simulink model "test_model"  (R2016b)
settings: Solver=VariableStepAuto  StartTime=0.0  StopTime=runtime  RelTol=1e-3
InitFcn:
  | clear mex
  | delete test_model_sfun.mexw64
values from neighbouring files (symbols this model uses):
  Delta_T = cell(1,4)    [modelParameters.m]
  F_D = 0    [modelParameters.m]
  g = 9.81    [modelParameters.m]
  Gamma_H = cell(1,4)    [modelParameters.m]
  have_motor_transient = 1    [modelParameters.m]
  height_controlled_o = (((Rm*If        + (((omega0_o * 2 * Rm * Kv * Kq      * Kd + 1)^2) - 1)/(4* Rm*Kv^2*Kq      * Kd))/Vb)*(Pmax - Pmin) + Pmin)    [modelParameters.m]
  i_0 = cell(1,4)    [modelParameters.m]
  If = 0.3836    [modelParameters.m]
  J = diag([ 0.0130 0.0140 0.0285 ])    [modelParameters.m]
  J_L = m_L/12*diag([y_L^2+z_L^2,x_L^2+z_L^2,x_L^2+y_L^2])    [modelParameters.m]
  J_r = cell(1,4)    [modelParameters.m]
  Jreq = 4.2012e-05    [modelParameters.m]
  Jxx = 0.0130    (= 0.013)    [modelParameters.m]
  Jyy = 0.0140    (= 0.014)    [modelParameters.m]
  Jzz = 0.0285    [modelParameters.m]
  K_d = cell(1,4)    [modelParameters.m]
  K_E = cell(1,4)    [modelParameters.m]
  K_H = cell(1,4)    [modelParameters.m]
  K_Q = cell(1,4)    [modelParameters.m]
  K_T = cell(1,4)    [modelParameters.m]
  K_V = cell(1,4)    [modelParameters.m]
  Kd = 1.4852e-07    [modelParameters.m]
  Ki_mahony = 0.001    [modelParameters.m]
  Kp_mahony = 0.4    [modelParameters.m]
  Kq = 96.3422    [modelParameters.m]
  Kt = 1.2007e-05    [modelParameters.m]
  Kv = 96.3422    [modelParameters.m]
  m = 1.216    [modelParameters.m]
  m_L = 0    [modelParameters.m]
  omega0_o = sqrt((m*g)/(4*Kt))    [modelParameters.m]
  omega1_o = sqrt((m*g)/(4*Kt))    [modelParameters.m]
  omega2_o = sqrt((m*g)/(4*Kt))    [modelParameters.m]
  omega3_o = sqrt((m*g)/(4*Kt))    [modelParameters.m]
  omega_0 = cell(1,4)    [modelParameters.m]
  p0 = 0    [modelParameters.m]
  p_0 = cell(1,4)    [modelParameters.m]
  p_max = cell(1,4)    [modelParameters.m]
  phi0 = 0    [modelParameters.m]
  pitch_o = 0    [modelParameters.m]
  pitchrate_o = 0    [modelParameters.m]
  Pmax = 1    [modelParameters.m]
  Pmin = 0    [modelParameters.m]
  psi0 = 0    [modelParameters.m]
  q0 = 0    [modelParameters.m]
  Q_D = 0    [modelParameters.m]
  r0 = 0    [modelParameters.m]
  R_m = cell(1,4)    [modelParameters.m]
  r_oc = [ 0 ; 0 ; 0 ]    [modelParameters.m]
  r_oL = [0; 0; 0]    [modelParameters.m]
  rhx = 0.16    [modelParameters.m]
  rhy = 0.16    [modelParameters.m]
  rhz = 0.03    [modelParameters.m]
  Rm = 0.235    [modelParameters.m]
  roll_o = 0    [modelParameters.m]
  rollrate_o = 0    [modelParameters.m]
  Tc = 0.04    [modelParameters.m]
  theta0 = 0    [modelParameters.m]
  Tq = 0.005    [modelParameters.m]
  u0 = 0    [modelParameters.m]
  v0 = 0    [modelParameters.m]
  Vb = 11.4    [modelParameters.m]
  w0 = 0    [modelParameters.m]
  x0 = 0    [modelParameters.m]
  x_controlled_o = 0    [modelParameters.m]
  x_o = 0    [modelParameters.m]
  x_vel_o = 0    [modelParameters.m]
  y0 = 0    [modelParameters.m]
  y_controlled_o = 0    [modelParameters.m]
  y_o = 0    [modelParameters.m]
  y_vel_o = 0    [modelParameters.m]
  yaw_controlled_o = 0    [modelParameters.m]
  yaw_o = 0    [modelParameters.m]
  yawrate_o = 0    [modelParameters.m]
  z0 = 0    [modelParameters.m]
  z_o = 0    [modelParameters.m]
  z_vel_o = 0    [modelParameters.m]
undefined symbols (not defined in the file or in its folder): Gamma_Omega, Gamma_T, Ki, Kp, r_h, slope, start, Ts, X0
libraries: simulink x16, Derivative x13, dsparch4 x3, vrlib x2
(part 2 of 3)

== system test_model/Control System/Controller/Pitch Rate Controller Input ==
  note: 1) Add Subsystem or Model blocks as valid variant choices. 2) You cannot connect blocks at this level. At simulation, connectivity is automatically determined, based on the active variant and port name matching.
  pitchrate_error_model : Inport
  pitchrate_model : Inport  Port=2
  Feedback : Subsystem  VariantControl=logAnalysisToggle==0
  pitchrate error : Subsystem  VariantControl=logAnalysisToggle==1
  pitchrate_error : Outport
  pitchrate : Outport  Port=2

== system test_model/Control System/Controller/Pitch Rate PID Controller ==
  pitchrate_error : Inport
  pitchrate : Inport  Port=2
  Add : Sum  Inputs=+-
  Discrete D Controller : Derivative/Discrete D Controller  Kd=Kd  a=a
  Discrete PI Controller : simulink/Continuous/PID Controller  Controller=PI  TimeDomain=Discrete-time  SampleTime=Ts  IntegratorMethod=Forward Euler  FilterMethod=Forward Euler  Form=Parallel  UseFilter=on  ControllerParametersSource=internal  P=Kp  I=Ki  D=0  N=100  InitialConditionSource=internal  InitialConditionForIntegrator=0  InitialConditionForFilter=0  ExternalReset=none  LimitOutput=off  UpperSaturationLimit=inf  LowerSaturationLimit=-inf  LinearizeAsGain=off  AntiWindupMode=none  Kb=1  TrackingMode=off  Kt=1  PParamMin=[]  PParamMax=[]  IParamMin=[]  IParamMax=[]  DParamMin=[]  DParamMax=[]  NParamMin=[]  NParamMax=[]  KbParamMin=[]  KbParamMax=[]  KtParamMin=[]  KtParamMax=[]  POutMin=[]  POutMax=[]  IOutMin=[]  IOutMax=[]  DOutMin=[]  DOutMax=[]  NOutMin=[]  NOutMax=[]  KbOutMin=[]  KbOutMax=[]  KtOutMin=[]  KtOutMax=[]  IntegratorOutMin=[]  IntegratorOutMax=[]  FilterOutMin=[]  FilterOutMax=[]  SumOutMin=[]  SumOutMax=[]  SumI1OutMin=[]  SumI1OutMax=[]  SumI2OutMin=[]  SumI2OutMax=[]  SumI3OutMin=[]  SumI3OutMax=[]  SumDOutMin=[]  SumDOutMax=[]  SaturationOutMin=[]  SaturationOutMax=[]  IntegratorContinuousStateAttributes=''  IntegratorStateMustResolveToSignalObject=off  IntegratorRTWStateStorageClass=Auto  FilterContinuousStateAttributes=''  FilterStateMustResolveToSignalObject=off  FilterRTWStateStorageClass=Auto  DifferentiatorICPrevScaledInput=0  DifferentiatorOutMin=[]  DifferentiatorOutMax=[]
  x_motor_command : Outport
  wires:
  pitchrate/1 -> Discrete D Controller/1
  pitchrate_error/1 -> Discrete PI Controller/1
  Discrete PI Controller/1 -> Add/1
  Discrete D Controller/1 -> Add/2
  Add/1 -> x_motor_command/1

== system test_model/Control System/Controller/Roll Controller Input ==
  note: 1) Add Subsystem or Model blocks as valid variant choices. 2) You cannot connect blocks at this level. At simulation, connectivity is automatically determined, based on the active variant and port name matching.
  roll_error_model : Inport
  roll_angle_model : Inport  Port=2
  Feedback : Subsystem  VariantControl=logAnalysisToggle==0
  roll error : Subsystem  VariantControl=logAnalysisToggle==1
  roll_error : Outport
  roll_angle : Outport  Port=2

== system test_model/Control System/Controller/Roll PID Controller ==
  roll_error : Inport
  roll_angle : Inport  Port=2
  Add : Sum  Inputs=+-
  Discrete D Controller : Derivative/Discrete D Controller  Kd=Kd  a=a
  Discrete PI Controller : simulink/Continuous/PID Controller  Controller=PI  TimeDomain=Discrete-time  SampleTime=Ts  IntegratorMethod=Forward Euler  FilterMethod=Forward Euler  Form=Parallel  UseFilter=on  ControllerParametersSource=internal  P=Kp  I=Ki  D=0  N=100  InitialConditionSource=internal  InitialConditionForIntegrator=0  InitialConditionForFilter=0  ExternalReset=none  LimitOutput=off  UpperSaturationLimit=inf  LowerSaturationLimit=-inf  LinearizeAsGain=off  AntiWindupMode=none  Kb=1  TrackingMode=off  Kt=1  PParamMin=[]  PParamMax=[]  IParamMin=[]  IParamMax=[]  DParamMin=[]  DParamMax=[]  NParamMin=[]  NParamMax=[]  KbParamMin=[]  KbParamMax=[]  KtParamMin=[]  KtParamMax=[]  POutMin=[]  POutMax=[]  IOutMin=[]  IOutMax=[]  DOutMin=[]  DOutMax=[]  NOutMin=[]  NOutMax=[]  KbOutMin=[]  KbOutMax=[]  KtOutMin=[]  KtOutMax=[]  IntegratorOutMin=[]  IntegratorOutMax=[]  FilterOutMin=[]  FilterOutMax=[]  SumOutMin=[]  SumOutMax=[]  SumI1OutMin=[]  SumI1OutMax=[]  SumI2OutMin=[]  SumI2OutMax=[]  SumI3OutMin=[]  SumI3OutMax=[]  SumDOutMin=[]  SumDOutMax=[]  SaturationOutMin=[]  SaturationOutMax=[]  IntegratorContinuousStateAttributes=''  IntegratorStateMustResolveToSignalObject=off  IntegratorRTWStateStorageClass=Auto  FilterContinuousStateAttributes=''  FilterStateMustResolveToSignalObject=off  FilterRTWStateStorageClass=Auto  DifferentiatorICPrevScaledInput=0  DifferentiatorOutMin=[]  DifferentiatorOutMax=[]
  rollrate_setpoint : Outport
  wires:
  roll_angle/1 -> Discrete D Controller/1
  roll_error/1 -> Discrete PI Controller/1
  Discrete PI Controller/1 -> Add/1
  Discrete D Controller/1 -> Add/2
  Add/1 -> rollrate_setpoint/1

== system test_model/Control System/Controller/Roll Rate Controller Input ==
  note: 1) Add Subsystem or Model blocks as valid variant choices. 2) You cannot connect blocks at this level. At simulation, connectivity is automatically determined, based on the active variant and port name matching.
  rollrate_error_model : Inport
  rollrate_model : Inport  Port=2
  Feedback : Subsystem  VariantControl=logAnalysisToggle==0
  rollrate error : Subsystem  VariantControl=logAnalysisToggle==1
  rollrate_error : Outport
  rollrate : Outport  Port=2

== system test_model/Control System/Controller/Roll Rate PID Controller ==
  rollrate_error : Inport
  rollrate : Inport  Port=2
  Add : Sum  Inputs=+-
  Discrete D Controller : Derivative/Discrete D Controller  Kd=Kd  a=a
  Discrete PI Controller : simulink/Continuous/PID Controller  Controller=PI  TimeDomain=Discrete-time  SampleTime=Ts  IntegratorMethod=Forward Euler  FilterMethod=Forward Euler  Form=Parallel  UseFilter=on  ControllerParametersSource=internal  P=Kp  I=Ki  D=0  N=100  InitialConditionSource=internal  InitialConditionForIntegrator=0  InitialConditionForFilter=0  ExternalReset=none  LimitOutput=off  UpperSaturationLimit=inf  LowerSaturationLimit=-inf  LinearizeAsGain=off  AntiWindupMode=none  Kb=1  TrackingMode=off  Kt=1  PParamMin=[]  PParamMax=[]  IParamMin=[]  IParamMax=[]  DParamMin=[]  DParamMax=[]  NParamMin=[]  NParamMax=[]  KbParamMin=[]  KbParamMax=[]  KtParamMin=[]  KtParamMax=[]  POutMin=[]  POutMax=[]  IOutMin=[]  IOutMax=[]  DOutMin=[]  DOutMax=[]  NOutMin=[]  NOutMax=[]  KbOutMin=[]  KbOutMax=[]  KtOutMin=[]  KtOutMax=[]  IntegratorOutMin=[]  IntegratorOutMax=[]  FilterOutMin=[]  FilterOutMax=[]  SumOutMin=[]  SumOutMax=[]  SumI1OutMin=[]  SumI1OutMax=[]  SumI2OutMin=[]  SumI2OutMax=[]  SumI3OutMin=[]  SumI3OutMax=[]  SumDOutMin=[]  SumDOutMax=[]  SaturationOutMin=[]  SaturationOutMax=[]  IntegratorContinuousStateAttributes=''  IntegratorStateMustResolveToSignalObject=off  IntegratorRTWStateStorageClass=Auto  FilterContinuousStateAttributes=''  FilterStateMustResolveToSignalObject=off  FilterRTWStateStorageClass=Auto  DifferentiatorICPrevScaledInput=0  DifferentiatorOutMin=[]  DifferentiatorOutMax=[]
  y_motor_command : Outport
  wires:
  rollrate/1 -> Discrete D Controller/1
  rollrate_error/1 -> Discrete PI Controller/1
  Discrete PI Controller/1 -> Add/1
  Discrete D Controller/1 -> Add/2
  Add/1 -> y_motor_command/1

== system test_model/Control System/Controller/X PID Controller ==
  x_error : Inport
  x_pos : Inport  Port=2
  Add : Sum  Inputs=+-
  Discrete D Controller : Derivative/Discrete D Controller  Kd=Kd  a=a
  Discrete PI Controller : simulink/Continuous/PID Controller  Controller=PI  TimeDomain=Discrete-time  SampleTime=Ts  IntegratorMethod=Forward Euler  FilterMethod=Forward Euler  Form=Parallel  UseFilter=on  ControllerParametersSource=internal  P=Kp  I=Ki  D=0  N=100  InitialConditionSource=internal  InitialConditionForIntegrator=0  InitialConditionForFilter=0  ExternalReset=none  LimitOutput=off  UpperSaturationLimit=inf  LowerSaturationLimit=-inf  LinearizeAsGain=off  AntiWindupMode=none  Kb=1  TrackingMode=off  Kt=1  PParamMin=[]  PParamMax=[]  IParamMin=[]  IParamMax=[]  DParamMin=[]  DParamMax=[]  NParamMin=[]  NParamMax=[]  KbParamMin=[]  KbParamMax=[]  KtParamMin=[]  KtParamMax=[]  POutMin=[]  POutMax=[]  IOutMin=[]  IOutMax=[]  DOutMin=[]  DOutMax=[]  NOutMin=[]  NOutMax=[]  KbOutMin=[]  KbOutMax=[]  KtOutMin=[]  KtOutMax=[]  IntegratorOutMin=[]  IntegratorOutMax=[]  FilterOutMin=[]  FilterOutMax=[]  SumOutMin=[]  SumOutMax=[]  SumI1OutMin=[]  SumI1OutMax=[]  SumI2OutMin=[]  SumI2OutMax=[]  SumI3OutMin=[]  SumI3OutMax=[]  SumDOutMin=[]  SumDOutMax=[]  SaturationOutMin=[]  SaturationOutMax=[]  IntegratorContinuousStateAttributes=''  IntegratorStateMustResolveToSignalObject=off  IntegratorRTWStateStorageClass=Auto  FilterContinuousStateAttributes=''  FilterStateMustResolveToSignalObject=off  FilterRTWStateStorageClass=Auto  DifferentiatorICPrevScaledInput=0  DifferentiatorOutMin=[]  DifferentiatorOutMax=[]
  pitch_setpoint : Outport
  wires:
  x_pos/1 -> Discrete D Controller/1
  x_error/1 -> Discrete PI Controller/1
  Discrete PI Controller/1 -> Add/1
  Discrete D Controller/1 -> Add/2
  Add/1 -> pitch_setpoint/1

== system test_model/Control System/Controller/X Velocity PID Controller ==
  x_vel_error : Inport
  x_vel : Inport  Port=2
  Add : Sum  Inputs=+-
  Discrete D Controller : Derivative/Discrete D Controller  Kd=Kd  a=a
  Discrete PI Controller : simulink/Continuous/PID Controller  Controller=PI  TimeDomain=Discrete-time  SampleTime=Ts  IntegratorMethod=Forward Euler  FilterMethod=Forward Euler  Form=Parallel  UseFilter=on  ControllerParametersSource=internal  P=Kp  I=Ki  D=0  N=100  InitialConditionSource=internal  InitialConditionForIntegrator=0  InitialConditionForFilter=0  ExternalReset=none  LimitOutput=off  UpperSaturationLimit=inf  LowerSaturationLimit=-inf  LinearizeAsGain=off  AntiWindupMode=none  Kb=1  TrackingMode=off  Kt=1  PParamMin=[]  PParamMax=[]  IParamMin=[]  IParamMax=[]  DParamMin=[]  DParamMax=[]  NParamMin=[]  NParamMax=[]  KbParamMin=[]  KbParamMax=[]  KtParamMin=[]  KtParamMax=[]  POutMin=[]  POutMax=[]  IOutMin=[]  IOutMax=[]  DOutMin=[]  DOutMax=[]  NOutMin=[]  NOutMax=[]  KbOutMin=[]  KbOutMax=[]  KtOutMin=[]  KtOutMax=[]  IntegratorOutMin=[]  IntegratorOutMax=[]  FilterOutMin=[]  FilterOutMax=[]  SumOutMin=[]  SumOutMax=[]  SumI1OutMin=[]  SumI1OutMax=[]  SumI2OutMin=[]  SumI2OutMax=[]  SumI3OutMin=[]  SumI3OutMax=[]  SumDOutMin=[]  SumDOutMax=[]  SaturationOutMin=[]  SaturationOutMax=[]  IntegratorContinuousStateAttributes=''  IntegratorStateMustResolveToSignalObject=off  IntegratorRTWStateStorageClass=Auto  FilterContinuousStateAttributes=''  FilterStateMustResolveToSignalObject=off  FilterRTWStateStorageClass=Auto  DifferentiatorICPrevScaledInput=0  DifferentiatorOutMin=[]  DifferentiatorOutMax=[]
  pitch_setpoint : Outport
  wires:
  x_vel/1 -> Discrete D Controller/1
  x_vel_error/1 -> Discrete PI Controller/1
  Discrete PI Controller/1 -> Add/1
  Discrete D Controller/1 -> Add/2
  Add/1 -> pitch_setpoint/1

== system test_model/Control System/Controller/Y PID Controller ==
  y_error : Inport
  y_pos : Inport  Port=2
  Add : Sum  Inputs=+-
  Discrete D Controller : Derivative/Discrete D Controller  Kd=Kd  a=a
  Discrete PI Controller : simulink/Continuous/PID Controller  Controller=PI  TimeDomain=Discrete-time  SampleTime=Ts  IntegratorMethod=Forward Euler  FilterMethod=Forward Euler  Form=Parallel  UseFilter=on  ControllerParametersSource=internal  P=Kp  I=Ki  D=0  N=100  InitialConditionSource=internal  InitialConditionForIntegrator=0  InitialConditionForFilter=0  ExternalReset=none  LimitOutput=off  UpperSaturationLimit=inf  LowerSaturationLimit=-inf  LinearizeAsGain=off  AntiWindupMode=none  Kb=1  TrackingMode=off  Kt=1  PParamMin=[]  PParamMax=[]  IParamMin=[]  IParamMax=[]  DParamMin=[]  DParamMax=[]  NParamMin=[]  NParamMax=[]  KbParamMin=[]  KbParamMax=[]  KtParamMin=[]  KtParamMax=[]  POutMin=[]  POutMax=[]  IOutMin=[]  IOutMax=[]  DOutMin=[]  DOutMax=[]  NOutMin=[]  NOutMax=[]  KbOutMin=[]  KbOutMax=[]  KtOutMin=[]  KtOutMax=[]  IntegratorOutMin=[]  IntegratorOutMax=[]  FilterOutMin=[]  FilterOutMax=[]  SumOutMin=[]  SumOutMax=[]  SumI1OutMin=[]  SumI1OutMax=[]  SumI2OutMin=[]  SumI2OutMax=[]  SumI3OutMin=[]  SumI3OutMax=[]  SumDOutMin=[]  SumDOutMax=[]  SaturationOutMin=[]  SaturationOutMax=[]  IntegratorContinuousStateAttributes=''  IntegratorStateMustResolveToSignalObject=off  IntegratorRTWStateStorageClass=Auto  FilterContinuousStateAttributes=''  FilterStateMustResolveToSignalObject=off  FilterRTWStateStorageClass=Auto  DifferentiatorICPrevScaledInput=0  DifferentiatorOutMin=[]  DifferentiatorOutMax=[]
  roll_setpoint : Outport
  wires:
  y_pos/1 -> Discrete D Controller/1
  y_error/1 -> Discrete PI Controller/1
  Discrete PI Controller/1 -> Add/1
  Discrete D Controller/1 -> Add/2
  Add/1 -> roll_setpoint/1

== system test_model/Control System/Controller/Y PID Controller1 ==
  y_error : Inport
  y_pos : Inport  Port=2
  Add : Sum  Inputs=+-
  Discrete D Controller : Derivative/Discrete D Controller  Kd=Kd  a=a
  Discrete PI Controller : simulink/Continuous/PID Controller  Controller=PI  TimeDomain=Discrete-time  SampleTime=Ts  IntegratorMethod=Forward Euler  FilterMethod=Forward Euler  Form=Parallel  UseFilter=on  ControllerParametersSource=internal  P=Kp  I=Ki  D=0  N=100  InitialConditionSource=internal  InitialConditionForIntegrator=0  InitialConditionForFilter=0  ExternalReset=none  LimitOutput=off  UpperSaturationLimit=inf  LowerSaturationLimit=-inf  LinearizeAsGain=off  AntiWindupMode=none  Kb=1  TrackingMode=off  Kt=1  PParamMin=[]  PParamMax=[]  IParamMin=[]  IParamMax=[]  DParamMin=[]  DParamMax=[]  NParamMin=[]  NParamMax=[]  KbParamMin=[]  KbParamMax=[]  KtParamMin=[]  KtParamMax=[]  POutMin=[]  POutMax=[]  IOutMin=[]  IOutMax=[]  DOutMin=[]  DOutMax=[]  NOutMin=[]  NOutMax=[]  KbOutMin=[]  KbOutMax=[]  KtOutMin=[]  KtOutMax=[]  IntegratorOutMin=[]  IntegratorOutMax=[]  FilterOutMin=[]  FilterOutMax=[]  SumOutMin=[]  SumOutMax=[]  SumI1OutMin=[]  SumI1OutMax=[]  SumI2OutMin=[]  SumI2OutMax=[]  SumI3OutMin=[]  SumI3OutMax=[]  SumDOutMin=[]  SumDOutMax=[]  SaturationOutMin=[]  SaturationOutMax=[]  IntegratorContinuousStateAttributes=''  IntegratorStateMustResolveToSignalObject=off  IntegratorRTWStateStorageClass=Auto  FilterContinuousStateAttributes=''  FilterStateMustResolveToSignalObject=off  FilterRTWStateStorageClass=Auto  DifferentiatorICPrevScaledInput=0  DifferentiatorOutMin=[]  DifferentiatorOutMax=[]
  y_vel_setpoint : Outport
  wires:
  y_pos/1 -> Discrete D Controller/1
  y_error/1 -> Discrete PI Controller/1
  Discrete PI Controller/1 -> Add/1
  Discrete D Controller/1 -> Add/2
  Add/1 -> y_vel_setpoint/1

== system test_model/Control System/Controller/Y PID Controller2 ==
  x_error : Inport
  x_pos : Inport  Port=2
  Add : Sum  Inputs=+-
  Discrete D Controller : Derivative/Discrete D Controller  Kd=Kd  a=a
  Discrete PI Controller : simulink/Continuous/PID Controller  Controller=PI  TimeDomain=Discrete-time  SampleTime=Ts  IntegratorMethod=Forward Euler  FilterMethod=Forward Euler  Form=Parallel  UseFilter=on  ControllerParametersSource=internal  P=Kp  I=Ki  D=0  N=100  InitialConditionSource=internal  InitialConditionForIntegrator=0  InitialConditionForFilter=0  ExternalReset=none  LimitOutput=off  UpperSaturationLimit=inf  LowerSaturationLimit=-inf  LinearizeAsGain=off  AntiWindupMode=none  Kb=1  TrackingMode=off  Kt=1  PParamMin=[]  PParamMax=[]  IParamMin=[]  IParamMax=[]  DParamMin=[]  DParamMax=[]  NParamMin=[]  NParamMax=[]  KbParamMin=[]  KbParamMax=[]  KtParamMin=[]  KtParamMax=[]  POutMin=[]  POutMax=[]  IOutMin=[]  IOutMax=[]  DOutMin=[]  DOutMax=[]  NOutMin=[]  NOutMax=[]  KbOutMin=[]  KbOutMax=[]  KtOutMin=[]  KtOutMax=[]  IntegratorOutMin=[]  IntegratorOutMax=[]  FilterOutMin=[]  FilterOutMax=[]  SumOutMin=[]  SumOutMax=[]  SumI1OutMin=[]  SumI1OutMax=[]  SumI2OutMin=[]  SumI2OutMax=[]  SumI3OutMin=[]  SumI3OutMax=[]  SumDOutMin=[]  SumDOutMax=[]  SaturationOutMin=[]  SaturationOutMax=[]  IntegratorContinuousStateAttributes=''  IntegratorStateMustResolveToSignalObject=off  IntegratorRTWStateStorageClass=Auto  FilterContinuousStateAttributes=''  FilterStateMustResolveToSignalObject=off  FilterRTWStateStorageClass=Auto  DifferentiatorICPrevScaledInput=0  DifferentiatorOutMin=[]  DifferentiatorOutMax=[]
  x_vel_setpoint : Outport
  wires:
  x_pos/1 -> Discrete D Controller/1
  x_error/1 -> Discrete PI Controller/1
  Discrete PI Controller/1 -> Add/1
  Discrete D Controller/1 -> Add/2
  Add/1 -> x_vel_setpoint/1

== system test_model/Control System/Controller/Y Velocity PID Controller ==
  y_error : Inport
  y_pos : Inport  Port=2
  Add : Sum  Inputs=+-
  Discrete D Controller : Derivative/Discrete D Controller  Kd=Kd  a=a
  Discrete PI Controller : simulink/Continuous/PID Controller  Controller=PI  TimeDomain=Discrete-time  SampleTime=Ts  IntegratorMethod=Forward Euler  FilterMethod=Forward Euler  Form=Parallel  UseFilter=on  ControllerParametersSource=internal  P=Kp  I=Ki  D=0  N=100  InitialConditionSource=internal  InitialConditionForIntegrator=0  InitialConditionForFilter=0  ExternalReset=none  LimitOutput=off  UpperSaturationLimit=inf  LowerSaturationLimit=-inf  LinearizeAsGain=off  AntiWindupMode=none  Kb=1  TrackingMode=off  Kt=1  PParamMin=[]  PParamMax=[]  IParamMin=[]  IParamMax=[]  DParamMin=[]  DParamMax=[]  NParamMin=[]  NParamMax=[]  KbParamMin=[]  KbParamMax=[]  KtParamMin=[]  KtParamMax=[]  POutMin=[]  POutMax=[]  IOutMin=[]  IOutMax=[]  DOutMin=[]  DOutMax=[]  NOutMin=[]  NOutMax=[]  KbOutMin=[]  KbOutMax=[]  KtOutMin=[]  KtOutMax=[]  IntegratorOutMin=[]  IntegratorOutMax=[]  FilterOutMin=[]  FilterOutMax=[]  SumOutMin=[]  SumOutMax=[]  SumI1OutMin=[]  SumI1OutMax=[]  SumI2OutMin=[]  SumI2OutMax=[]  SumI3OutMin=[]  SumI3OutMax=[]  SumDOutMin=[]  SumDOutMax=[]  SaturationOutMin=[]  SaturationOutMax=[]  IntegratorContinuousStateAttributes=''  IntegratorStateMustResolveToSignalObject=off  IntegratorRTWStateStorageClass=Auto  FilterContinuousStateAttributes=''  FilterStateMustResolveToSignalObject=off  FilterRTWStateStorageClass=Auto  DifferentiatorICPrevScaledInput=0  DifferentiatorOutMin=[]  DifferentiatorOutMax=[]
  roll_setpoint : Outport
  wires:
  y_pos/1 -> Discrete D Controller/1
  y_error/1 -> Discrete PI Controller/1
  Discrete PI Controller/1 -> Add/1
  Discrete D Controller/1 -> Add/2
  Add/1 -> roll_setpoint/1

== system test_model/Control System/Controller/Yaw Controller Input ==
  note: 1) Add Subsystem or Model blocks as valid variant choices. 2) You cannot connect blocks at this level. At simulation, connectivity is automatically determined, based on the active variant and port name matching.
  yaw_error_model : Inport
  yaw_angle_model : Inport  Port=2
  Feedback : Subsystem  VariantControl=logAnalysisToggle==0
  yaw error : Subsystem  VariantControl=logAnalysisToggle==1
  yaw_error : Outport
  yaw_angle : Outport  Port=2

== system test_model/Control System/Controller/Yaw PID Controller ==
  yaw_error : Inport
  yaw_angle : Inport  Port=2
  Add : Sum  Inputs=+-
  Discrete D Controller : Derivative/Discrete D Controller  Kd=Kd  a=a
  Discrete PI Controller : simulink/Continuous/PID Controller  Controller=PI  TimeDomain=Discrete-time  SampleTime=Ts  IntegratorMethod=Forward Euler  FilterMethod=Forward Euler  Form=Parallel  UseFilter=on  ControllerParametersSource=internal  P=Kp  I=Ki  D=0  N=100  InitialConditionSource=internal  InitialConditionForIntegrator=0  InitialConditionForFilter=0  ExternalReset=none  LimitOutput=off  UpperSaturationLimit=inf  LowerSaturationLimit=-inf  LinearizeAsGain=off  AntiWindupMode=none  Kb=1  TrackingMode=off  Kt=1  PParamMin=[]  PParamMax=[]  IParamMin=[]  IParamMax=[]  DParamMin=[]  DParamMax=[]  NParamMin=[]  NParamMax=[]  KbParamMin=[]  KbParamMax=[]  KtParamMin=[]  KtParamMax=[]  POutMin=[]  POutMax=[]  IOutMin=[]  IOutMax=[]  DOutMin=[]  DOutMax=[]  NOutMin=[]  NOutMax=[]  KbOutMin=[]  KbOutMax=[]  KtOutMin=[]  KtOutMax=[]  IntegratorOutMin=[]  IntegratorOutMax=[]  FilterOutMin=[]  FilterOutMax=[]  SumOutMin=[]  SumOutMax=[]  SumI1OutMin=[]  SumI1OutMax=[]  SumI2OutMin=[]  SumI2OutMax=[]  SumI3OutMin=[]  SumI3OutMax=[]  SumDOutMin=[]  SumDOutMax=[]  SaturationOutMin=[]  SaturationOutMax=[]  IntegratorContinuousStateAttributes=''  IntegratorStateMustResolveToSignalObject=off  IntegratorRTWStateStorageClass=Auto  FilterContinuousStateAttributes=''  FilterStateMustResolveToSignalObject=off  FilterRTWStateStorageClass=Auto  DifferentiatorICPrevScaledInput=0  DifferentiatorOutMin=[]  DifferentiatorOutMax=[]
  yawrate_setpoint : Outport
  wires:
  yaw_angle/1 -> Discrete D Controller/1
  yaw_error/1 -> Discrete PI Controller/1
  Discrete PI Controller/1 -> Add/1
  Discrete D Controller/1 -> Add/2
  Add/1 -> yawrate_setpoint/1

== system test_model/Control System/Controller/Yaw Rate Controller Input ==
  note: 1) Add Subsystem or Model blocks as valid variant choices. 2) You cannot connect blocks at this level. At simulation, connectivity is automatically determined, based on the active variant and port name matching.
  yawrate_error_model : Inport
  yawrate_model : Inport  Port=2
  Feedback : Subsystem  VariantControl=logAnalysisToggle==0
  yawrate error : Subsystem  VariantControl=logAnalysisToggle==1
  yawrate_error : Outport
  yawrate : Outport  Port=2

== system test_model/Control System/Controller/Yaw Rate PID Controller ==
  yawrate_error : Inport
  yawrate : Inport  Port=2
  Add : Sum  Inputs=+-
  Discrete D Controller : Derivative/Discrete D Controller  Kd=Kd  a=a
  Discrete PI Controller : simulink/Continuous/PID Controller  Controller=PI  TimeDomain=Discrete-time  SampleTime=Ts  IntegratorMethod=Forward Euler  FilterMethod=Forward Euler  Form=Parallel  UseFilter=on  ControllerParametersSource=internal  P=Kp  I=Ki  D=0  N=100  InitialConditionSource=internal  InitialConditionForIntegrator=0  InitialConditionForFilter=0  ExternalReset=none  LimitOutput=off  UpperSaturationLimit=inf  LowerSaturationLimit=-inf  LinearizeAsGain=off  AntiWindupMode=none  Kb=1  TrackingMode=off  Kt=1  PParamMin=[]  PParamMax=[]  IParamMin=[]  IParamMax=[]  DParamMin=[]  DParamMax=[]  NParamMin=[]  NParamMax=[]  KbParamMin=[]  KbParamMax=[]  KtParamMin=[]  KtParamMax=[]  POutMin=[]  POutMax=[]  IOutMin=[]  IOutMax=[]  DOutMin=[]  DOutMax=[]  NOutMin=[]  NOutMax=[]  KbOutMin=[]  KbOutMax=[]  KtOutMin=[]  KtOutMax=[]  IntegratorOutMin=[]  IntegratorOutMax=[]  FilterOutMin=[]  FilterOutMax=[]  SumOutMin=[]  SumOutMax=[]  SumI1OutMin=[]  SumI1OutMax=[]  SumI2OutMin=[]  SumI2OutMax=[]  SumI3OutMin=[]  SumI3OutMax=[]  SumDOutMin=[]  SumDOutMax=[]  SaturationOutMin=[]  SaturationOutMax=[]  IntegratorContinuousStateAttributes=''  IntegratorStateMustResolveToSignalObject=off  IntegratorRTWStateStorageClass=Auto  FilterContinuousStateAttributes=''  FilterStateMustResolveToSignalObject=off  FilterRTWStateStorageClass=Auto  DifferentiatorICPrevScaledInput=0  DifferentiatorOutMin=[]  DifferentiatorOutMax=[]
  yaw_motor_command : Outport
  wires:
  yawrate/1 -> Discrete D Controller/1
  yawrate_error/1 -> Discrete PI Controller/1
  Discrete PI Controller/1 -> Add/1
  Discrete D Controller/1 -> Add/2
  Add/1 -> yaw_motor_command/1

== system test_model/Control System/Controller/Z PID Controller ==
  z_error : Inport
  z_pos : Inport  Port=2
  Add : Sum  Inputs=+-
  Discrete D Controller : Derivative/Discrete D Controller  Kd=Kd  a=a
  Discrete PI Controller : simulink/Continuous/PID Controller  Controller=PI  TimeDomain=Discrete-time  SampleTime=Ts  IntegratorMethod=Forward Euler  FilterMethod=Forward Euler  Form=Parallel  UseFilter=on  ControllerParametersSource=internal  P=Kp  I=Ki  D=0  N=100  InitialConditionSource=internal  InitialConditionForIntegrator=0  InitialConditionForFilter=0  ExternalReset=none  LimitOutput=off  UpperSaturationLimit=inf  LowerSaturationLimit=-inf  LinearizeAsGain=off  AntiWindupMode=none  Kb=1  TrackingMode=off  Kt=1  PParamMin=[]  PParamMax=[]  IParamMin=[]  IParamMax=[]  DParamMin=[]  DParamMax=[]  NParamMin=[]  NParamMax=[]  KbParamMin=[]  KbParamMax=[]  KtParamMin=[]  KtParamMax=[]  POutMin=[]  POutMax=[]  IOutMin=[]  IOutMax=[]  DOutMin=[]  DOutMax=[]  NOutMin=[]  NOutMax=[]  KbOutMin=[]  KbOutMax=[]  KtOutMin=[]  KtOutMax=[]  IntegratorOutMin=[]  IntegratorOutMax=[]  FilterOutMin=[]  FilterOutMax=[]  SumOutMin=[]  SumOutMax=[]  SumI1OutMin=[]  SumI1OutMax=[]  SumI2OutMin=[]  SumI2OutMax=[]  SumI3OutMin=[]  SumI3OutMax=[]  SumDOutMin=[]  SumDOutMax=[]  SaturationOutMin=[]  SaturationOutMax=[]  IntegratorContinuousStateAttributes=''  IntegratorStateMustResolveToSignalObject=off  IntegratorRTWStateStorageClass=Auto  FilterContinuousStateAttributes=''  FilterStateMustResolveToSignalObject=off  FilterRTWStateStorageClass=Auto  DifferentiatorICPrevScaledInput=0  DifferentiatorOutMin=[]  DifferentiatorOutMax=[]
  z_motor_command : Outport
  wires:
  z_pos/1 -> Discrete D Controller/1
  z_error/1 -> Discrete PI Controller/1
  Discrete PI Controller/1 -> Add/1
  Discrete D Controller/1 -> Add/2
  Add/1 -> z_motor_command/1

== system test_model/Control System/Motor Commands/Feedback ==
  z_command_model : Inport
  z_command : Outport
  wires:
  z_command_model/1 -> z_command/1

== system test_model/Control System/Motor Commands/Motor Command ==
  From Workspace5 : FromWorkspace  VariableName=motor_commands  SampleTime=Tq
  z_command : Outport
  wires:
  From Workspace5/1 -> z_command/1

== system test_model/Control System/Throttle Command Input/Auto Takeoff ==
  height_controlled_o : Constant  Value=0.45  SampleTime=Tc
  z_command : Outport
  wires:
  height_controlled_o/1 -> z_command/1

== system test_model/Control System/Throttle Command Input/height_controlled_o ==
  height_controlled_o : Constant  Value=height_controlled_o  SampleTime=Tc
  z_command : Outport
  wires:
  height_controlled_o/1 -> z_command/1

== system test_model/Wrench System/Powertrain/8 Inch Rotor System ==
  M : Inport
  Lambda : Inport  Port=2
  8 Inch Rotor 1 : Subsystem
  8 Inch Rotor 2 : Subsystem
  8 Inch Rotor 3 : Subsystem
  8 Inch Rotor 4 : Subsystem
  Bus Creator : BusCreator  Inputs=8
  Bus Selector : BusSelector  OutputSignals=signal1.alpha_1,signal1.omega_1
  Bus Selector1 : BusSelector  OutputSignals=signal2.alpha_2,signal2.omega_2
  Bus Selector2 : BusSelector  OutputSignals=signal3.alpha_3,signal3.omega_3
  Bus Selector3 : BusSelector  OutputSignals=signal4.alpha_4,signal4.omega_4
  Bus Selector{4..7} (4 alike) : BusSelector  OutputSignals=v_o,Omega
  W_r : Outport
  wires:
  8 Inch Rotor 4/1(F) -> Bus Creator/7  "F_r_4"
  8 Inch Rotor 3/2(Q) -> Bus Creator/6  "Q_r_3"
  8 Inch Rotor 3/1(F) -> Bus Creator/5  "F_r_3"
  8 Inch Rotor 2/2(Q) -> Bus Creator/4  "Q_r_2"
  8 Inch Rotor 2/1(F) -> Bus Creator/3  "F_r_2"
  8 Inch Rotor 4/2(Q) -> Bus Creator/8  "Q_r_4"
  8 Inch Rotor 1/2(Q) -> Bus Creator/2  "Q_r_1"
  8 Inch Rotor 1/1(F) -> Bus Creator/1  "F_r_1"
  Bus Creator/1 -> W_r/1
  Bus Selector/1 -> 8 Inch Rotor 1/1(alpha)  "<alpha_1>"
  Bus Selector/2 -> 8 Inch Rotor 1/2(omega)  "<omega_1>"
  Bus Selector4/1 -> 8 Inch Rotor 1/3(v)  "<v_o>"
  Bus Selector4/2 -> 8 Inch Rotor 1/4(Omega)  "<Omega>"
  Bus Selector1/1 -> 8 Inch Rotor 2/1(alpha)  "<alpha_2>"
  Bus Selector1/2 -> 8 Inch Rotor 2/2(omega)  "<omega_2>"
  Bus Selector5/1 -> 8 Inch Rotor 2/3(v)  "<v_o>"
  Bus Selector5/2 -> 8 Inch Rotor 2/4(Omega)  "<Omega>"
  Bus Selector2/1 -> 8 Inch Rotor 3/1(alpha)  "<alpha_3>"
  Bus Selector2/2 -> 8 Inch Rotor 3/2(omega)  "<omega_3>"
  Bus Selector7/1 -> 8 Inch Rotor 3/3(v)  "<v_o>"
  Bus Selector7/2 -> 8 Inch Rotor 3/4(Omega)  "<Omega>"
  Bus Selector3/1 -> 8 Inch Rotor 4/1(alpha)  "<alpha_4>"
  Bus Selector3/2 -> 8 Inch Rotor 4/2(omega)  "<omega_4>"
  Bus Selector6/1 -> 8 Inch Rotor 4/3(v)  "<v_o>"
  Bus Selector6/2 -> 8 Inch Rotor 4/4(Omega)  "<Omega>"
  Lambda/1 -> Bus Selector4/1, Bus Selector5/1, Bus Selector7/1, Bus Selector6/1
  M/1 -> Bus Selector/1, Bus Selector1/1, Bus Selector2/1, Bus Selector3/1

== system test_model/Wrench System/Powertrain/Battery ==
  Ramp : Subsystem
  V : Outport
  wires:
  Ramp/1(Out1) -> V/1

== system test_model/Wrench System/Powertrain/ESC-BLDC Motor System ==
  P : Inport
  V_b : Inport  Port=2
  Bus Creator{,1..3} (4 alike) : BusCreator  Inputs=2
  Bus Creator4 : BusCreator  Inputs=4
  Demux : Demux
  ESC and BLDC Motor 1 : Subsystem
  ESC and BLDC Motor 2 : Subsystem
  ESC and BLDC Motor 3 : Subsystem
  ESC and BLDC Motor 4 : Subsystem
  M : Outport
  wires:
  Bus Creator4/1 -> M/1
  V_b/1 -> ESC and BLDC Motor 4/2(V_b), ESC and BLDC Motor 3/2(V_b), ESC and BLDC Motor 2/2(V_b), ESC and BLDC Motor 1/2(V_b)
  ESC and BLDC Motor 1/2(omega) -> Bus Creator/2  "omega_1"
  ESC and BLDC Motor 1/1(alpha) -> Bus Creator/1  "alpha_1"
  ESC and BLDC Motor 2/1(alpha) -> Bus Creator1/1  "alpha_2"
  ESC and BLDC Motor 2/2(omega) -> Bus Creator1/2  "omega_2"
  ESC and BLDC Motor 3/1(alpha) -> Bus Creator2/1  "alpha_3"
  ESC and BLDC Motor 3/2(omega) -> Bus Creator2/2  "omega_3"
  ESC and BLDC Motor 4/1(alpha) -> Bus Creator3/1  "alpha_4"
  ESC and BLDC Motor 4/2(omega) -> Bus Creator3/2  "omega_4"
  Bus Creator/1 -> Bus Creator4/1
  Bus Creator1/1 -> Bus Creator4/2
  Bus Creator3/1 -> Bus Creator4/4
  Bus Creator2/1 -> Bus Creator4/3
  P/1 -> Demux/1
  Demux/1 -> ESC and BLDC Motor 2/1(p)
  Demux/2 -> ESC and BLDC Motor 1/1(p)
  Demux/3 -> ESC and BLDC Motor 3/1(p)
  Demux/4 -> ESC and BLDC Motor 4/1(p)

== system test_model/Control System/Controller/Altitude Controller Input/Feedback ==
  z_error_model : Inport
  z_position_model : Inport  Port=2
  z_error : Outport
  z_position : Outport  Port=2
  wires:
  z_error_model/1 -> z_error/1
  z_position_model/1 -> z_position/1

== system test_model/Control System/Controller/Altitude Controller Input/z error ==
  From Workspace1 : FromWorkspace  VariableName=z_position  SampleTime=Tc  Interpolate=off  OutputAfterFinalValue=Holding final value
  From Workspace6 : FromWorkspace  VariableName=z_error  SampleTime=Tc  Interpolate=off  OutputAfterFinalValue=Holding final value
  z_error : Outport
  z_position : Outport  Port=2
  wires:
  From Workspace6/1 -> z_error/1
  From Workspace1/1 -> z_position/1

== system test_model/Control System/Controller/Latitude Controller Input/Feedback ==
  x_error_model : Inport
  x_position_model : Inport  Port=2
  x_error : Outport
  x_position : Outport  Port=2
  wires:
  x_error_model/1 -> x_error/1
  x_position_model/1 -> x_position/1

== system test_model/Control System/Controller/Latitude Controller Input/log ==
  From Workspace : FromWorkspace  VariableName=x_error  SampleTime=Tc  Interpolate=off  OutputAfterFinalValue=Holding final value
  From Workspace1 : FromWorkspace  VariableName=x_position  SampleTime=Tc  Interpolate=off  OutputAfterFinalValue=Holding final value
  x_error : Outport
  x_position : Outport  Port=2
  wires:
  From Workspace/1 -> x_error/1
  From Workspace1/1 -> x_position/1

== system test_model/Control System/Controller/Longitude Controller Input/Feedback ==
  y_error_model : Inport
  y_position_model : Inport  Port=2
  y_error : Outport
  y_position : Outport  Port=2
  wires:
  y_error_model/1 -> y_error/1
  y_position_model/1 -> y_position/1

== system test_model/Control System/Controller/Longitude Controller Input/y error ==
  From Workspace1 : FromWorkspace  VariableName=y_position  SampleTime=Tc  Interpolate=off  OutputAfterFinalValue=Holding final value
  From Workspace3 : FromWorkspace  VariableName=y_error  SampleTime=Tc  Interpolate=off  OutputAfterFinalValue=Holding final value
  y_error : Outport
  y_position : Outport  Port=2
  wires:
  From Workspace3/1 -> y_error/1
  From Workspace1/1 -> y_position/1

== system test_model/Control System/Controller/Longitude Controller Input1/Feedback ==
  y_vel_error_model : Inport
  y_vel_model : Inport  Port=2
  y_vel_error : Outport
  y_vel : Outport  Port=2
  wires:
  y_vel_error_model/1 -> y_vel_error/1
  y_vel_model/1 -> y_vel/1

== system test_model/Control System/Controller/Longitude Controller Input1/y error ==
  From Workspace1 : FromWorkspace  VariableName=y_vel  SampleTime=Tc  Interpolate=off  OutputAfterFinalValue=Holding final value
  From Workspace3 : FromWorkspace  VariableName=y_vel_error  SampleTime=Tc  Interpolate=off  OutputAfterFinalValue=Holding final value
  y_vel_error : Outport
  y_vel : Outport  Port=2
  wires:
  From Workspace3/1 -> y_vel_error/1
  From Workspace1/1 -> y_vel/1

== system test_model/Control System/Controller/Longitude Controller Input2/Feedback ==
  x_vel_error_model : Inport
  x_vel_model : Inport  Port=2
  x_vel_error : Outport
  x_vel : Outport  Port=2
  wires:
  x_vel_error_model/1 -> x_vel_error/1
  x_vel_model/1 -> x_vel/1

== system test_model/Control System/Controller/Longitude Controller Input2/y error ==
  From Workspace1 : FromWorkspace  VariableName=x_vel  SampleTime=Tc  Interpolate=off  OutputAfterFinalValue=Holding final value
  From Workspace3 : FromWorkspace  VariableName=x_vel_error  SampleTime=Tc  Interpolate=off  OutputAfterFinalValue=Holding final value
  x_vel_error : Outport
  x_vel : Outport  Port=2
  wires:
  From Workspace3/1 -> x_vel_error/1
  From Workspace1/1 -> x_vel/1

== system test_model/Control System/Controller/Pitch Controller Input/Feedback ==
  pitch_error_model : Inport
  pitch_angle_model : Inport  Port=2
  pitch_error : Outport
  pitch_angle : Outport  Port=2
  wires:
  pitch_error_model/1 -> pitch_error/1
  pitch_angle_model/1 -> pitch_angle/1

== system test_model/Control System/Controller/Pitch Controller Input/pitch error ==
  From Workspace : FromWorkspace  VariableName=pitch_error  SampleTime=Tq  Interpolate=off  OutputAfterFinalValue=Holding final value
  From Workspace1 : FromWorkspace  VariableName=pitch_angle  SampleTime=Tq  Interpolate=off  OutputAfterFinalValue=Holding final value
  pitch_error : Outport
  pitch_angle : Outport  Port=2
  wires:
  From Workspace/1 -> pitch_error/1
  From Workspace1/1 -> pitch_angle/1

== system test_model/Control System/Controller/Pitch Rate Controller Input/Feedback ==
  pitchrate_error_model : Inport
  pitchrate_model : Inport  Port=2
  pitchrate_error : Outport
  pitchrate : Outport  Port=2
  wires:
  pitchrate_error_model/1 -> pitchrate_error/1
  pitchrate_model/1 -> pitchrate/1

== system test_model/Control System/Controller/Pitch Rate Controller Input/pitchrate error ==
  From Workspace1 : FromWorkspace  VariableName=pitchrate  SampleTime=Tq  Interpolate=off  OutputAfterFinalValue=Holding final value
  From Workspace2 : FromWorkspace  VariableName=pitchrate_error  SampleTime=Tq  Interpolate=off  OutputAfterFinalValue=Holding final value
  pitchrate_error : Outport
  pitchrate : Outport  Port=2
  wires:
  From Workspace2/1 -> pitchrate_error/1
  From Workspace1/1 -> pitchrate/1

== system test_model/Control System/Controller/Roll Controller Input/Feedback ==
  roll_error_model : Inport
  roll_angle_model : Inport  Port=2
  roll_error : Outport
  roll_angle : Outport  Port=2
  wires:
  roll_error_model/1 -> roll_error/1
  roll_angle_model/1 -> roll_angle/1

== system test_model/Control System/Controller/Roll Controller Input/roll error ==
  From Workspace1 : FromWorkspace  VariableName=roll_angle  SampleTime=Tq  Interpolate=off  OutputAfterFinalValue=Holding final value
  From Workspace4 : FromWorkspace  VariableName=roll_error  SampleTime=Tq  Interpolate=off  OutputAfterFinalValue=Holding final value
  roll_error : Outport
  roll_angle : Outport  Port=2
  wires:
  From Workspace4/1 -> roll_error/1
  From Workspace1/1 -> roll_angle/1

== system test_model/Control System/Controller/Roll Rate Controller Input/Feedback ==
  rollrate_error_model : Inport
  rollrate_model : Inport  Port=2
  rollrate_error : Outport
  rollrate : Outport  Port=2
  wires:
  rollrate_error_model/1 -> rollrate_error/1
  rollrate_model/1 -> rollrate/1

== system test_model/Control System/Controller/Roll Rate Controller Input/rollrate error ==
  From Workspace1 : FromWorkspace  VariableName=rollrate  SampleTime=Tq  Interpolate=off  OutputAfterFinalValue=Holding final value
  From Workspace5 : FromWorkspace  VariableName=rollrate_error  SampleTime=Tq  Interpolate=off  OutputAfterFinalValue=Holding final value
  rollrate_error : Outport
  rollrate : Outport  Port=2
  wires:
  From Workspace5/1 -> rollrate_error/1
  From Workspace1/1 -> rollrate/1

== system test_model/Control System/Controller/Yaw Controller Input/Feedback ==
  yaw_error_model : Inport
  yaw_angle_model : Inport  Port=2
  yaw_error : Outport
  yaw_angle : Outport  Port=2
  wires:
  yaw_error_model/1 -> yaw_error/1
  yaw_angle_model/1 -> yaw_angle/1

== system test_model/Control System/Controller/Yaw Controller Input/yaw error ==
  From Workspace1 : FromWorkspace  VariableName=yaw_angle  SampleTime=Tc  Interpolate=off  OutputAfterFinalValue=Holding final value
  From Workspace7 : FromWorkspace  VariableName=yaw_error  SampleTime=Tc  Interpolate=off  OutputAfterFinalValue=Holding final value
  yaw_error : Outport
  yaw_angle : Outport  Port=2
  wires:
  From Workspace7/1 -> yaw_error/1
  From Workspace1/1 -> yaw_angle/1

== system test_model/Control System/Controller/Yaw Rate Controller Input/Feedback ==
  yawrate_error_model : Inport
  yawrate_model : Inport  Port=2
  yawrate_error : Outport
  yawrate : Outport  Port=2
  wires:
  yawrate_error_model/1 -> yawrate_error/1
  yawrate_model/1 -> yawrate/1

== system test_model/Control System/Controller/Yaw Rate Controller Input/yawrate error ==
  From Workspace1 : FromWorkspace  VariableName=yawrate  SampleTime=Tq  Interpolate=off  OutputAfterFinalValue=Holding final value
  From Workspace8 : FromWorkspace  VariableName=yawrate_error  SampleTime=Tq  Interpolate=off  OutputAfterFinalValue=Holding final value
  yawrate_error : Outport
  yawrate : Outport  Port=2
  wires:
  From Workspace8/1 -> yawrate_error/1
  From Workspace1/1 -> yawrate/1

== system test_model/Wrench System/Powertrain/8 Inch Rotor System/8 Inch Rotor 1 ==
  alpha : Inport
  omega : Inport  Port=2
  v : Inport  Port=3
  Omega : Inport  Port=4
  8 Inch Rotor : MATLAB Function
  Delta_T : Constant  Value=Delta_T
  Gamma_H : Constant  Value=Gamma_H
  Gamma_Omega : Constant  Value=Gamma_Omega
  Gamma_T : Constant  Value=Gamma_T
  J_r : Constant  Value=J_r
  K_H : Constant  Value=K_H
  K_T : Constant  Value=K_T
  K_d : Constant  Value=K_d
  r_h : Constant  Value=r_h
  F : Outport
  Q : Outport  Port=2
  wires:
  8 Inch Rotor/2(Q) -> Q/1
  8 Inch Rotor/1(F) -> F/1
  Omega/1 -> 8 Inch Rotor/4(Omega)
  v/1 -> 8 Inch Rotor/3(v)
  K_T/1 -> 8 Inch Rotor/5(K_T)
  Gamma_Omega/1 -> 8 Inch Rotor/12(Gamma_Omega)
  Gamma_H/1 -> 8 Inch Rotor/11(Gamma_H)
  Gamma_T/1 -> 8 Inch Rotor/10(Gamma_T)
  Delta_T/1 -> 8 Inch Rotor/9(Delta_T)
  r_h/1 -> 8 Inch Rotor/8(r_h)
  K_d/1 -> 8 Inch Rotor/7(K_d)
  K_H/1 -> 8 Inch Rotor/6(K_H)
  omega/1 -> 8 Inch Rotor/1(omega)
  alpha/1 -> 8 Inch Rotor/2(alpha)
  J_r/1 -> 8 Inch Rotor/13(J_r)

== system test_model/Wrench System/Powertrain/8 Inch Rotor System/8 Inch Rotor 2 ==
  alpha : Inport
  omega : Inport  Port=2
  v : Inport  Port=3
  Omega : Inport  Port=4
  8 Inch Rotor : MATLAB Function
  Delta_T : Constant  Value=Delta_T
  Gamma_H : Constant  Value=Gamma_H
  Gamma_Omega : Constant  Value=Gamma_Omega
  Gamma_T : Constant  Value=Gamma_T
  J_r : Constant  Value=J_r
  K_H : Constant  Value=K_H
  K_T : Constant  Value=K_T
  K_d : Constant  Value=K_d
  r_h : Constant  Value=r_h
  F : Outport
  Q : Outport  Port=2
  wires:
  8 Inch Rotor/2(Q) -> Q/1
  8 Inch Rotor/1(F) -> F/1
  Omega/1 -> 8 Inch Rotor/4(Omega)
  v/1 -> 8 Inch Rotor/3(v)
  K_T/1 -> 8 Inch Rotor/5(K_T)
  Gamma_Omega/1 -> 8 Inch Rotor/12(Gamma_Omega)
  Gamma_H/1 -> 8 Inch Rotor/11(Gamma_H)
  Gamma_T/1 -> 8 Inch Rotor/10(Gamma_T)
  Delta_T/1 -> 8 Inch Rotor/9(Delta_T)
  r_h/1 -> 8 Inch Rotor/8(r_h)
  K_d/1 -> 8 Inch Rotor/7(K_d)
  K_H/1 -> 8 Inch Rotor/6(K_H)
  omega/1 -> 8 Inch Rotor/1(omega)
  alpha/1 -> 8 Inch Rotor/2(alpha)
  J_r/1 -> 8 Inch Rotor/13(J_r)

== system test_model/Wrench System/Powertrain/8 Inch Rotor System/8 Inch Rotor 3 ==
  alpha : Inport
  omega : Inport  Port=2
  v : Inport  Port=3
  Omega : Inport  Port=4
  8 Inch Rotor : MATLAB Function
  Delta_T : Constant  Value=Delta_T
  Gamma_H : Constant  Value=Gamma_H
  Gamma_Omega : Constant  Value=Gamma_Omega
  Gamma_T : Constant  Value=Gamma_T
  J_r : Constant  Value=J_r
  K_H : Constant  Value=K_H
  K_T : Constant  Value=K_T
  K_d : Constant  Value=K_d
  r_h : Constant  Value=r_h
  F : Outport
  Q : Outport  Port=2
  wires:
  8 Inch Rotor/2(Q) -> Q/1
  8 Inch Rotor/1(F) -> F/1
  Omega/1 -> 8 Inch Rotor/4(Omega)
  v/1 -> 8 Inch Rotor/3(v)
  K_T/1 -> 8 Inch Rotor/5(K_T)
  Gamma_Omega/1 -> 8 Inch Rotor/12(Gamma_Omega)
  Gamma_H/1 -> 8 Inch Rotor/11(Gamma_H)
  Gamma_T/1 -> 8 Inch Rotor/10(Gamma_T)
  Delta_T/1 -> 8 Inch Rotor/9(Delta_T)
  r_h/1 -> 8 Inch Rotor/8(r_h)
  K_d/1 -> 8 Inch Rotor/7(K_d)
  K_H/1 -> 8 Inch Rotor/6(K_H)
  omega/1 -> 8 Inch Rotor/1(omega)
  alpha/1 -> 8 Inch Rotor/2(alpha)
  J_r/1 -> 8 Inch Rotor/13(J_r)

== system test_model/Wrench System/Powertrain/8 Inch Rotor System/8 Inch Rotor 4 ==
  alpha : Inport
  omega : Inport  Port=2
  v : Inport  Port=3
  Omega : Inport  Port=4
  8 Inch Rotor : MATLAB Function
  Delta_T : Constant  Value=Delta_T
  Gamma_H : Constant  Value=Gamma_H
  Gamma_Omega : Constant  Value=Gamma_Omega
  Gamma_T : Constant  Value=Gamma_T
  J_r : Constant  Value=J_r
  K_H : Constant  Value=K_H
  K_T : Constant  Value=K_T
  K_d : Constant  Value=K_d
  r_h : Constant  Value=r_h
  F : Outport
  Q : Outport  Port=2
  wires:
  8 Inch Rotor/2(Q) -> Q/1
  8 Inch Rotor/1(F) -> F/1
  Omega/1 -> 8 Inch Rotor/4(Omega)
  v/1 -> 8 Inch Rotor/3(v)
  K_T/1 -> 8 Inch Rotor/5(K_T)
  Gamma_Omega/1 -> 8 Inch Rotor/12(Gamma_Omega)
  Gamma_H/1 -> 8 Inch Rotor/11(Gamma_H)
  Gamma_T/1 -> 8 Inch Rotor/10(Gamma_T)
  Delta_T/1 -> 8 Inch Rotor/9(Delta_T)
  r_h/1 -> 8 Inch Rotor/8(r_h)
  K_d/1 -> 8 Inch Rotor/7(K_d)
  K_H/1 -> 8 Inch Rotor/6(K_H)
  omega/1 -> 8 Inch Rotor/1(omega)
  alpha/1 -> 8 Inch Rotor/2(alpha)
  J_r/1 -> 8 Inch Rotor/13(J_r)

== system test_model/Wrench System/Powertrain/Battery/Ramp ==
  Clock : Clock
  Constant : Constant  DisableCoverage=on  Value=start  OutDataTypeStr=Inherit: Inherit via back propagation
  Constant1 : Constant  DisableCoverage=on  Value=X0  OutDataTypeStr=Inherit: Inherit via back propagation
  Output : Sum  Inputs=|++
  Product : Product  DisableCoverage=on
  Step : Step  DisableCoverage=on  Time=start  After=slope  SampleTime=0
  Sum : Sum  DisableCoverage=on  Inputs=|+-
  Out1 : Outport
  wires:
  Clock/1 -> Sum/1
  Constant/1 -> Sum/2
  Sum/1 -> Product/2
  Output/1 -> Out1/1
  Constant1/1 -> Output/2
  Product/1 -> Output/1
  Step/1 -> Product/1

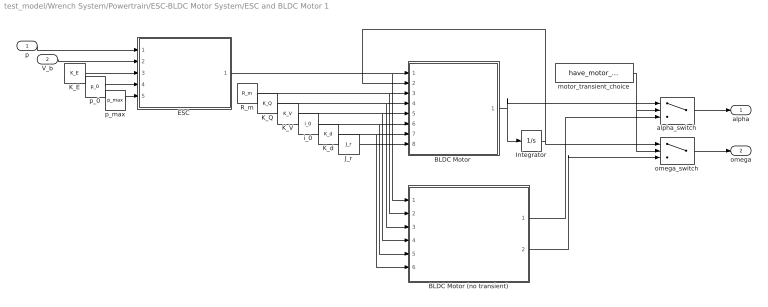
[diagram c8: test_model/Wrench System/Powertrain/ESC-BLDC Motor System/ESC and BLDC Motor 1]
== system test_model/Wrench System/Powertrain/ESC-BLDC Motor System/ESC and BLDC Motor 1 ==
  p : Inport
  V_b : Inport  Port=2
  "BLDC Motor " : MATLAB Function  TreatAsAtomicUnit=on
  BLDC Motor (no transient) : MATLAB Function  TreatAsAtomicUnit=on
  "ESC " : MATLAB Function  TreatAsAtomicUnit=on
  Integrator : Integrator  InitialCondition=omega_0  ContinuousStateAttributes='omega'
  J_r : Constant  Value=J_r
  K_E : Constant  Value=K_E
  K_Q : Constant  Value=K_Q
  K_V : Constant  Value=K_V
  K_d : Constant  Value=K_d
  R_m : Constant  Value=R_m
  alpha_switch : Switch  Criteria=u2 ~= 0
  i_0 : Constant  Value=i_0
  motor_transient_choice : Constant  Value=have_motor_transient
  omega_switch : Switch  Criteria=u2 ~= 0
  p_0 : Constant  Value=p_0
  p_max : Constant  Value=p_max
  alpha : Outport
  omega : Outport  Port=2
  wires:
  motor_transient_choice/1 -> omega_switch/2, alpha_switch/2
  omega_switch/1 -> omega/1
  alpha_switch/1 -> alpha/1
  BLDC Motor (no transient)/2(omega) -> omega_switch/3
  BLDC Motor (no transient)/1(alpha) -> alpha_switch/3
  Integrator/1 -> omega_switch/1, "BLDC Motor "/2(omega)
  "ESC "/1(V) -> BLDC Motor (no transient)/1(V), "BLDC Motor "/1(V)
  p/1 -> "ESC "/1(p)
  V_b/1 -> "ESC "/2(V_b)
  K_E/1 -> "ESC "/3(K_E)
  p_0/1 -> "ESC "/4(p_0)
  p_max/1 -> "ESC "/5(p_max)
  J_r/1 -> "BLDC Motor "/8(J_r)
  R_m/1 -> BLDC Motor (no transient)/2(R_m), "BLDC Motor "/3(R_m)
  "BLDC Motor "/1(alpha) -> alpha_switch/1, Integrator/1
  K_Q/1 -> BLDC Motor (no transient)/3(K_Q), "BLDC Motor "/4(K_Q)
  K_V/1 -> BLDC Motor (no transient)/4(K_V), "BLDC Motor "/5(K_V)
  i_0/1 -> BLDC Motor (no transient)/5(i_0), "BLDC Motor "/6(i_0)
  K_d/1 -> BLDC Motor (no transient)/6(K_d), "BLDC Motor "/7(K_d)
